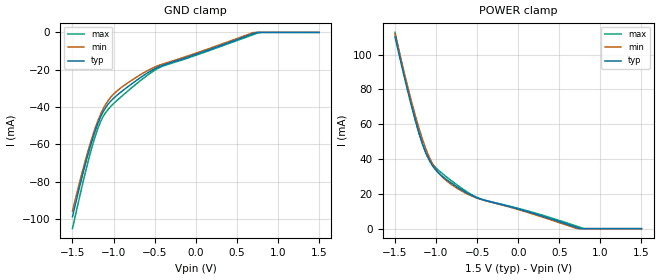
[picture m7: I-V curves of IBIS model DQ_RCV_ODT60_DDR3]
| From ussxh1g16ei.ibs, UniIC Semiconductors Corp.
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|   Model DQ_RCV_ODT60_DDR3
[Model] DQ_RCV_ODT60_DDR3
Model_type Input
Vinl =  0.615V
Vinh =  0.885V
C_comp   1.232pF   1.219pF   1.235pF
[Model Spec]
Vinh   0.885V   0.847V   0.922V
Vinl   0.615V   0.577V   0.652V
[Temperature Range]   25.000   95.000   -40.000
[Voltage Range]   1.500V   1.425V   1.575V
[GND_clamp]
|Voltage   I(typ)   I(min)   I(max)
-1.5V     -98.81mA   -95.83mA   -105.2mA
-1.376V   -76.25mA   -74.04mA   -81.11mA
-1.283V   -61.14mA   -59.44mA   -64.75mA
-1.221V   -52.48mA   -51.01mA   -55.36mA
-1.159V   -45.46mA   -44.01mA   -47.99mA
-1.097V   -40.36mA   -38.66mA   -43.02mA
-1.004V   -35.48mA   -33.3mA    -38.37mA
-663mV    -23.95mA   -22.42mA   -25.5mA
-415mV    -17.83mA   -17.18mA   -18.37mA
701mV     -713.4uA   -113.1uA   -1.179mA
763mV     0A         0A         -189.1uA
1.5V      0A         0A         0A
[POWER_clamp]
|Voltage   I(typ)   I(min)   I(max)
-1.5V     110.3mA    111.9mA    112.8mA
-1.29V    68.86mA    71.51mA    69.62mA
-1.166V   48.85mA    51.47mA    48.76mA
-1.104V   41.37mA    43.45mA    41.55mA
-1.042V   36.07mA    37.2mA     36.99mA
-949mV    31.13mA    30.93mA    32.68mA
-856mV    27.66mA    26.9mA     29.11mA
-639mV    20.97mA    20.4mA     21.66mA
-453mV    16.93mA    16.81mA    17.06mA
725mV     470.7uA    0A         1.192mA
818mV     0A         0A         0A
1.5V      0A         0A         0A
